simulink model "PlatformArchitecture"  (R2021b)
settings: Solver=VariableStepAuto  StartTime=0.0  StopTime=10.0  RelTol=1e-3

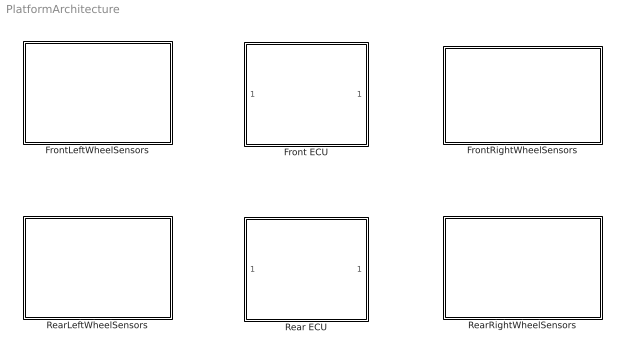
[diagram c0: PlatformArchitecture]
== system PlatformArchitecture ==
  Front ECU : ModelReference  ModelNameDialog=ECU  SimulationMode=Normal  ModelReferenceVersion=1.8
  FrontLeftWheelSensors : Subsystem
  FrontRightWheelSensors : Subsystem
  Rear ECU : ModelReference  ModelNameDialog=ECU  SimulationMode=Normal  ModelReferenceVersion=1.8
  RearLeftWheelSensors : Subsystem
  RearRightWheelSensors : Subsystem

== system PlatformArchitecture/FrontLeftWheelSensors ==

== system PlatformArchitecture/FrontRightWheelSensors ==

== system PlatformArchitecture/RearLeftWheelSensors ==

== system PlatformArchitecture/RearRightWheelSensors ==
